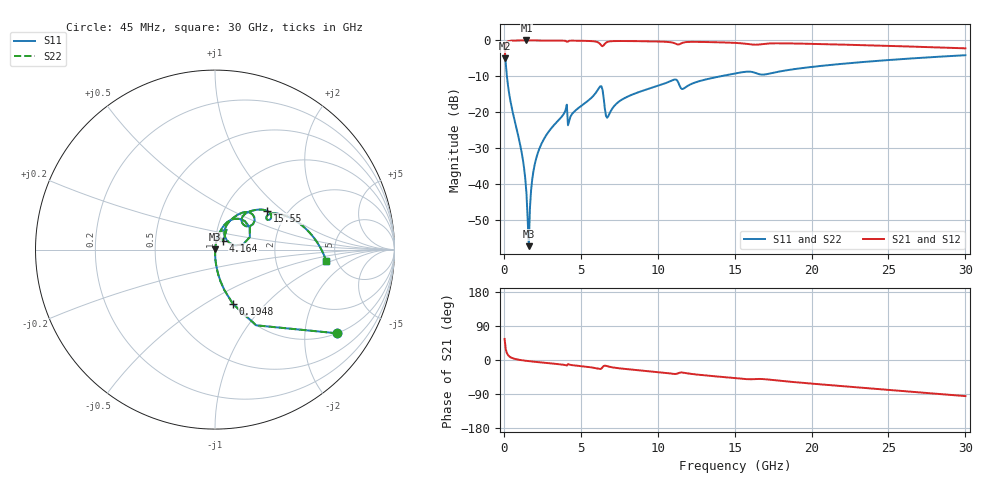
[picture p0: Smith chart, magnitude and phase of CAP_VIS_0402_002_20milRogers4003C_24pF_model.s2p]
! S-parameter model data by Modelithics Inc.  support@modelithics.com  813-866-6335  Tampa FL USA
! S-Parameter data specifications:
! Substrate: 20-mil Rogers 4003C, substrate thickness, H=0.508mm, Dielectric constant, Er=3.75
! PCB Mounting Pad Footprint: Pad width, PadW=0.50mm , Pad length, PadL=0.50mm , Pad gap, PadG (edge-to-edge)=0.40mm , Reference planes=1.4mm apart
! Created Wed Nov 18 12:53:09 2015
# hz S ma R 50
! 2 Port Network Data from SP1.SP block
! freq  magS11  angS11  magS21  angS21  magS12  angS12  magS22  angS22
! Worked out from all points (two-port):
!   401 points, 45 MHz to 30 GHz, reference 50 ohm
!   highest |S21| = -0.01 dB at 1.468 GHz (marker M1); lowest = -5.0 dB at 45 MHz (marker M2)
!   |S21| within 3 dB of the highest: 83.43 MHz to end of sweep
!   lowest |S11| = -57.3 dB at 1.618 GHz (marker M3), VSWR 1.00, Z = 50.1 + j0.0745 ohm
!   |S11| at or under -10 dB: 195 MHz to 14.06 GHz (13.86 GHz wide, 195 % of centre)
!   |S22| runs from -57.3 to -1.7 dB; largest |S21 - S12| = 0
!   S11 on the Smith chart (normalised r, x): 45 MHz: 1.00, -2.92; 194.8 MHz: 1.00, -0.67; 4.164 GHz: 1.09, +0.10; 15.55 GHz: 1.59, +0.78; 30 GHz: 4.12, -0.84
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4.5e7  0.8259 -34.4  0.5636 55.6  0.5636 55.6  0.8259 -34.4
1.94775e8  0.3166 -71.8  0.9482 18.1  0.9482 18.1  0.3166 -71.8
4.194375e8  0.145 -82.2  0.9888 7.6  0.9888 7.6  0.145 -82.2
1.2432e9  0.02122 -88.4  0.9988 -1.1  0.9988 -1.1  0.02122 -88.4
1.467862e9  0.007334 -84.0  0.9989 -2.3  0.9989 -2.3  0.007334 -84.0
1.617638e9  0.001372 32.8  0.9988 -3.0  0.9988 -3.0  0.001372 32.8
1.992075e9  0.01835 81.4  0.9985 -4.7  0.9985 -4.7  0.01835 81.4
2.366512e9  0.03358 81.4  0.998 -6.3  0.998 -6.3  0.03358 81.4
3.93915e9  0.09912 74.5  0.9906 -12.9  0.9906 -12.9  0.09912 74.5
4.163812e9  0.06592 46.4  0.9627 -10.8  0.9627 -10.8  0.06592 46.4
5.062462e9  0.1244 72.0  0.9886 -16.4  0.9886 -16.4  0.1244 72.0
6.260662e9  0.2298 43.9  0.8897 -23.8  0.8897 -23.8  0.2298 43.9
6.784875e9  0.08829 49.2  0.961 -17.1  0.961 -17.1  0.08829 49.2
7.758412e9  0.154 64.4  0.9811 -23.1  0.9811 -23.1  0.154 64.4
1.007992e10  0.2361 56.3  0.965 -32.2  0.965 -32.2  0.2361 56.3
1.112835e10  0.2864 43.1  0.9088 -36.8  0.9088 -36.8  0.2864 43.1
1.165256e10  0.2121 44.3  0.9325 -33.3  0.9325 -33.3  0.2121 44.3
1.50225e10  0.3467 39.9  0.9241 -47.9  0.9241 -47.9  0.3467 39.9
1.554671e10  0.3624 36.3  0.9075 -49.8  0.9075 -49.8  0.3624 36.3
2.003996e10  0.4285 26.6  0.8953 -62.4  0.8953 -62.4  0.4285 26.6
2.505742e10  0.5345 10.3  0.8387 -79.1  0.8387 -79.1  0.5345 10.3
3e10  0.6226 -5.8  0.7758 -95.3  0.7758 -95.3  0.6226 -5.8
